FUNCTION "DIVE" : VOID
TITLE =
VERSION : 0.1


VAR_TEMP
  zero : BOOL ;
END_VAR
BEGIN
NETWORK
TITLE =Produzione in corso
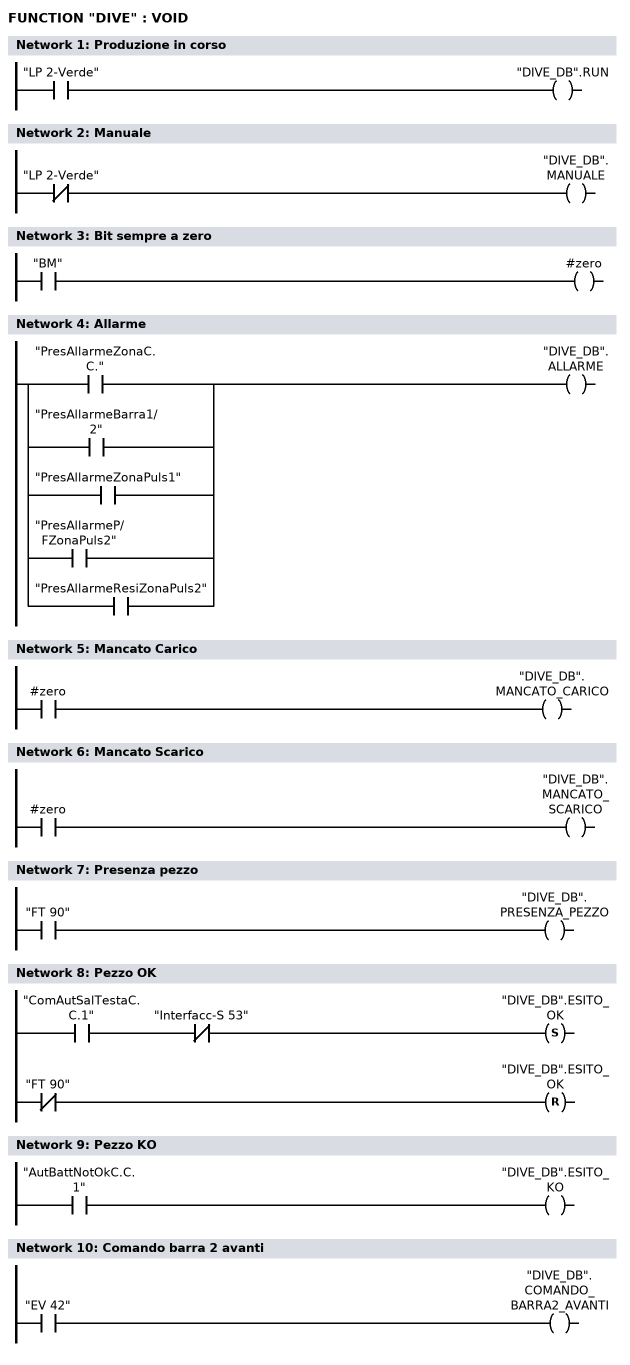
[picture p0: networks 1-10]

      U     "LP 2-Verde";
      =     "DIVE_DB".RUN;
NETWORK
TITLE =Manuale

      UN    "LP 2-Verde";
      =     "DIVE_DB".MANUALE;
NETWORK
TITLE =Bit sempre a zero

      U     "BM";
      =     #zero;
NETWORK
TITLE =Allarme

      O     "PresAllarmeZonaC.C.";
      O     "PresAllarmeBarra1/2";
      O     "PresAllarmeZonaPuls1";
      O     "PresAllarmeP/FZonaPuls2";
      O     "PresAllarmeResiZonaPuls2";
      =     "DIVE_DB".ALLARME;
NETWORK
TITLE =Mancato Carico

      U     #zero;
      =     "DIVE_DB".MANCATO_CARICO;
NETWORK
TITLE =Mancato Scarico

      U     #zero;
      =     "DIVE_DB".MANCATO_SCARICO;
NETWORK
TITLE =Presenza pezzo

      U     "FT 90";
      =     "DIVE_DB".PRESENZA_PEZZO;
NETWORK
TITLE =Pezzo OK

      U     "ComAutSalTestaC.C.1";
      UN    "Interfacc-S 53";
      S     "DIVE_DB".ESITO_OK;
      UN    "FT 90";
      R     "DIVE_DB".ESITO_OK;
      NOP   0;
NETWORK
TITLE =Pezzo KO

      U     "AutBattNotOkC.C.1";
      =     "DIVE_DB".ESITO_KO;
NETWORK
TITLE =Comando barra 2 avanti

      U     "EV 42";
      =     "DIVE_DB".COMANDO_BARRA2_AVANTI;
NETWORK
TITLE =Fine Lavoro

      U(    ;
      U(    ;
      O     "FineCicloAutZonaC.C.";
      ON    "BM";
      )     ;
      U     "ComAutSalTestaC.C.1";
      S     "M6.3";
      UN    "FT 90";
      R     "M6.3";
      U     "M6.3";
      )     ;
      L     S5T#500MS;
      SE    T     15;
      NOP   0;
      NOP   0;
      NOP   0;
      U     T     15;
      =     "DIVE_DB".FINE_LAVORO;
NETWORK
TITLE =Inizio Pallet
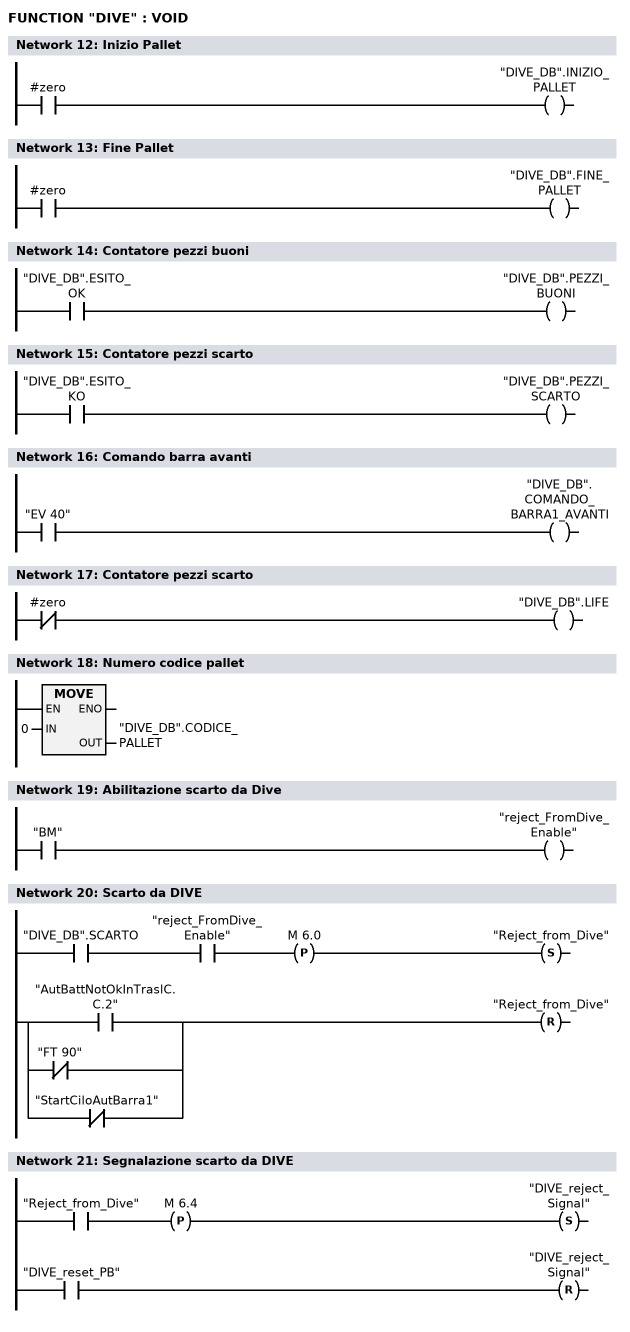
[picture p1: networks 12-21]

      U     #zero;
      =     "DIVE_DB".INIZIO_PALLET;
NETWORK
TITLE =Fine Pallet

      U     #zero;
      =     "DIVE_DB".FINE_PALLET;
NETWORK
TITLE =Contatore pezzi buoni

      U     "DIVE_DB".ESITO_OK;
      =     "DIVE_DB".PEZZI_BUONI;
NETWORK
TITLE =Contatore pezzi scarto

      U     "DIVE_DB".ESITO_KO;
      =     "DIVE_DB".PEZZI_SCARTO;
NETWORK
TITLE =Comando barra avanti

      U     "EV 40";
      =     "DIVE_DB".COMANDO_BARRA1_AVANTI;
NETWORK
TITLE =Contatore pezzi scarto

      UN    #zero;
      =     "DIVE_DB".LIFE;
NETWORK
TITLE =Numero codice pallet

      L     0;
      T     "DIVE_DB".CODICE_PALLET;
      NOP   0;
NETWORK
TITLE =Abilitazione scarto da Dive

      U     "BM";
      =     "reject_FromDive_Enable";
NETWORK
TITLE =Scarto da DIVE

      U     "DIVE_DB".SCARTO;
      U     "reject_FromDive_Enable";
      FP    M      6.0;
      S     "Reject_from_Dive";
      U(    ;
      O     "AutBattNotOkInTraslC.C.2";
      ON    "FT 90";
      ON    "StartCiloAutBarra1";
      )     ;
      R     "Reject_from_Dive";
      NOP   0;
NETWORK
TITLE =Segnalazione scarto da DIVE

      U     "Reject_from_Dive";
      FP    M      6.4;
      S     "DIVE_reject_Signal";
      U     "DIVE_reset_PB";
      R     "DIVE_reject_Signal";
      NOP   0;
END_FUNCTION

